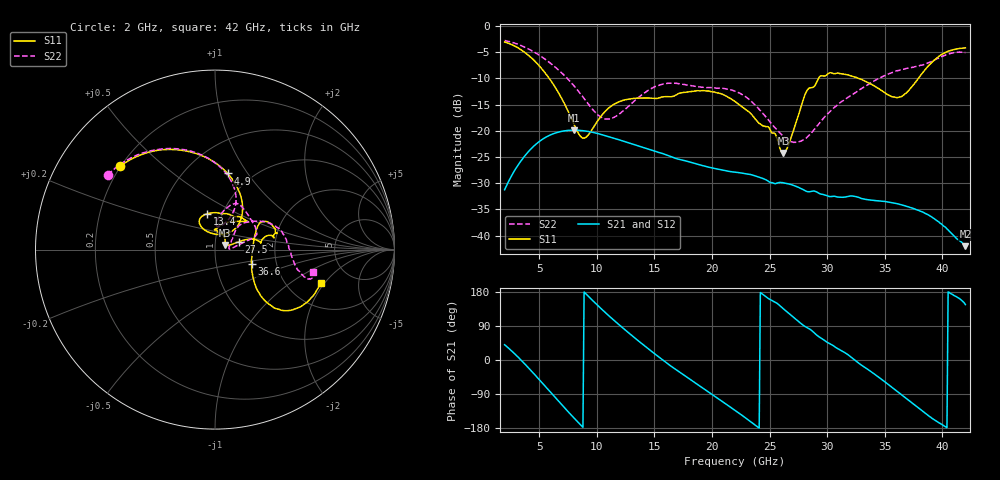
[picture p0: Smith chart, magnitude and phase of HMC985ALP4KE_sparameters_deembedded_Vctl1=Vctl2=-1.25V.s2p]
!s2p File: Measurements: S11, S21, S12, S22
# GHz S dB R 50.0
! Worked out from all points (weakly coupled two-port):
!   401 points, 2 GHz to 42 GHz, reference 50 ohm
!   highest |S21| = -19.86 dB at 8 GHz (marker M1); lowest = -42.0 dB at 42 GHz (marker M2)
!   lowest |S11| = -24.2 dB at 26.2 GHz (marker M3), VSWR 1.13, Z = 55.9 + j2.88 ohm
!   |S11| at or under -10 dB: 5.877 GHz to 29.25 GHz (23.37 GHz wide, 133 % of centre); 32.74 GHz to 37.91 GHz (5.176 GHz wide, 14.7 % of centre)
!   |S22| runs from -22.2 to -2.8 dB; largest |S21 - S12| = 0.00019
!   S11 on the Smith chart (normalised r, x): 2 GHz: 0.20, +0.36; 4.9 GHz: 0.78, +0.81; 13.4 GHz: 0.85, +0.35; 27.5 GHz: 1.30, +0.12; 36.6 GHz: 1.49, -0.25; 42 GHz: 3.04, -1.85
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2  -3.05 138.6  -31.24 40.3  -31.25 40.3  -2.75 145.1
3.4  -4.50 111.0  -25.80 0.6  -25.80 0.6  -3.70 122.2
4.9  -7.33 80.6  -22.22 -48.2  -22.22 -48.2  -5.41 98.7
6.2  -11.03 56.8  -20.57 -92.6  -20.58 -92.6  -7.48 80.7
8  -18.63 51.8  -19.86 -152.3  -19.87 -152.3  -11.35 65.1
8.7  -21.28 75.4  -19.95 -174.4  -19.95 -174.4  -13.26 64.1
10.8  -16.13 121.2  -20.95 123.6  -20.95 123.6  -17.74 81.8
13.4  -13.78 102.6  -22.72 55.7  -22.73 55.7  -14.04 81.0
15.4  -13.71 75.9  -24.14 7.8  -24.14 7.8  -11.29 68.6
18.9  -12.37 40.3  -26.46 -67.8  -26.47 -67.8  -11.61 41.9
22  -14.39 55.4  -27.88 -132.7  -27.89 -132.7  -12.43 18.6
24.9  -19.25 87.3  -29.62 162.1  -29.62 162.1  -17.94 10.7
26.2  -24.21 24.6  -29.92 135.2  -29.93 135.2  -21.07 3.0
27.5  -17.08 18.1  -30.77 101.8  -30.78 101.8  -22.12 6.9
28.2  -12.51 13.1  -31.54 86.2  -31.55 86.2  -21.33 17.1
28.7  -11.74 8.4  -31.51 76.6  -31.51 76.6  -20.21 24.8
31.1  -9.07 20.0  -32.66 27.0  -32.66 27.0  -14.68 44.8
33.3  -10.52 30.8  -33.06 -20.0  -33.07 -20.1  -11.52 36.5
35.4  -13.24 10.0  -33.62 -66.7  -33.62 -66.8  -9.09 23.1
36.6  -13.22 -21.2  -34.21 -95.1  -34.22 -95.1  -8.25 14.1
39.6  -5.98 -42.4  -37.24 -163.6  -37.23 -163.7  -6.20 -15.1
42  -4.16 -17.6  -42.00 146.2  -41.99 146.3  -5.05 -13.0
